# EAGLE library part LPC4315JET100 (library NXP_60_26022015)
32-bit ARM Cortex-M4/M0 MCU; up to 1 MB flash and 136 kB SRAM; Ethernet, two High-speed USB, LCD, EMC The LPC435x/3x/2x/1x are ARM Cortex-M4 based microcontrollers for embedded applications which include an ARM Cortex-M0 coprocessor, up to 1 MB of flash and 136 kB of on-chip SRAM, 16 kB of EEPROM memory, a quad SPI Flash Interface (SPIFI), advanced configurable peripherals such as the State Configurable Timer (SCT) and the Serial General Purpose I/O (SGPIO) interface, two High-speed USB controllers, Ethernet, LCD, an external memory controller, and multiple digital and analog peripherals. The LPC435x/3x/2x/1x operate at CPU frequencies of up to 204 MHz. The ARM Cortex-M4 is a next generation 32-bit core that offers system enhancements such as low power consumption, enhanced debug features, and a high level of support block integration. The ARM Cortex-M4 CPU incorporates a 3-stage pipeline, uses a Harvard architecture with separate local instruction and data buses as well as a third bus for peripherals, and includes an internal prefetch unit that supports speculative branching. The ARM Cortex-M4 supports single-cycle digital signal processing and SIMD instructions. A hardware floating-point unit is integrated in the core. The ARM Cortex-M0 coprocessor is an energy-efficient and easy-to-use 32-bit core which is upward code- and tool-compatible with the Cortex-M4 core. The Cortex-M0 coprocessor, designed as a replacement for existing 8/16-bit microcontrollers, offers up to 204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
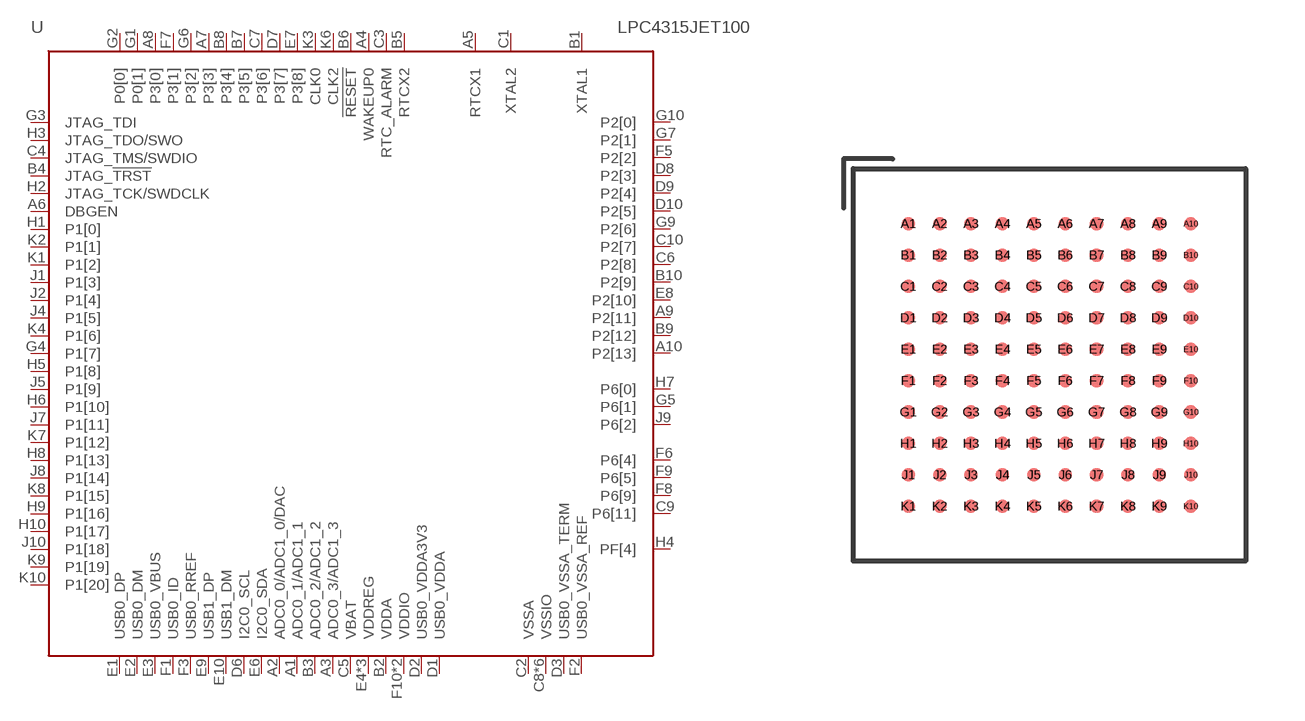
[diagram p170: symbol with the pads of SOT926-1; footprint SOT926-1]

Designator prefix U

## LPC4315JET100  [SOT926-1]
A1  ADC0_1/ADC1_1  in
A2  ADC0_0/ADC1_0/DAC  in
A3  ADC0_3/ADC1_3  in
A4  WAKEUP0  in
A5  RTCX1  in
A6  DBGEN  in
A7  P3[3]
A8  P3[0]
A9  P2[11]
A10  P2[13]
B1  XTAL1  in
B2  VDDA  pwr
B3  ADC0_2/ADC1_2  in
B4  JTAG_!TRST  in
B5  RTCX2  out
B6  !RESET!  in
B7  P3[5]
B8  P3[4]
B9  P2[12]
B10  P2[9]
C1  XTAL2  out
C2  VSSA  pwr
C3  RTC_ALARM  out
C4  JTAG_TMS/SWDIO  in
C5  VBAT  pwr
C6  P2[8]
C7  P3[6]
C8  VSSIO  pwr
C9  P6[11]
C10  P2[7]
D1  USB0_VDDA  pwr
D2  USB0_VDDA3V3  pwr
D3  USB0_VSSA_TERM  pwr
D4  VSSIO  pwr
D5  VSSIO  pwr
D6  I2C0_SCL
D7  P3[7]
D8  P2[3]
D9  P2[4]
D10  P2[5]
E1  USB0_DP
E2  USB0_DM
E3  USB0_VBUS
E4  VDDREG  pwr
E5  VDDREG  pwr
E6  I2C0_SDA
E7  P3[8]
E8  P2[10]
E9  USB1_DP
E10  USB1_DM
F1  USB0_ID  in
F2  USB0_VSSA_REF  pwr
F3  USB0_RREF  pas
F4  VDDREG  pwr
F5  P2[2]
F6  P6[4]
F7  P3[1]
F8  P6[9]
F9  P6[5]
F10  VDDIO  pwr
G1  P0[1]
G2  P0[0]
G3  JTAG_TDI  in
G4  P1[7]
G5  P6[1]
G6  P3[2]
G7  P2[1]
G8  VSSIO  pwr
G9  P2[6]
G10  P2[0]
H1  P1[0]
H2  JTAG_TCK/SWDCLK  in
H3  JTAG_TDO/SWO  out
H4  PF[4]
H5  P1[8]
H6  P1[10]
H7  P6[0]
H8  P1[13]
H9  P1[16]
H10  P1[17]
J1  P1[3]
J2  P1[4]
J3  VSSIO  pwr
J4  P1[5]
J5  P1[9]
J6  VSSIO  pwr
J7  P1[11]
J8  P1[14]
J9  P6[2]
J10  P1[18]
K1  P1[2]
K2  P1[1]
K3  CLK0
K4  P1[6]
K5  VDDIO  pwr
K6  CLK2
K7  P1[12]
K8  P1[15]
K9  P1[19]
K10  P1[20]

## Footprint SOT926-1 (pad centres in mm)
SOT926-1 TFBGA100: plastic thin fine-pitch ball grid array package; 100 balls; body 9 x 9 x 0.7 mm JEDEC: -- IEC: --
smd 0.35 x 0.35: A1 -3.6,3.6; A2 -2.8,3.6; A3 -2,3.6; A4 -1.2,3.6; A5 -0.4,3.6; A6 0.4,3.6; A7 1.2,3.6; A8 2,3.6; A9 2.8,3.6; A10 3.6,3.6; B1 -3.6,2.8; B2 -2.8,2.8; B3 -2,2.8; B4 -1.2,2.8; B5 -0.4,2.8; B6 0.4,2.8; B7 1.2,2.8; B8 2,2.8; B9 2.8,2.8; B10 3.6,2.8; C1 -3.6,2; C2 -2.8,2; C3 -2,2; C4 -1.2,2; C5 -0.4,2; C6 0.4,2; C7 1.2,2; C8 2,2; C9 2.8,2; C10 3.6,2; D1 -3.6,1.2; D2 -2.8,1.2; D3 -2,1.2; D4 -1.2,1.2; D5 -0.4,1.2; D6 0.4,1.2; D7 1.2,1.2; D8 2,1.2; D9 2.8,1.2; D10 3.6,1.2; E1 -3.6,0.4; E2 -2.8,0.4; E3 -2,0.4; E4 -1.2,0.4; E5 -0.4,0.4; E6 0.4,0.4; E7 1.2,0.4; E8 2,0.4; E9 2.8,0.4; E10 3.6,0.4; F1 -3.6,-0.4; F2 -2.8,-0.4; F3 -2,-0.4; F4 -1.2,-0.4; F5 -0.4,-0.4; F6 0.4,-0.4; F7 1.2,-0.4; F8 2,-0.4; F9 2.8,-0.4; F10 3.6,-0.4; G1 -3.6,-1.2; G2 -2.8,-1.2; G3 -2,-1.2; G4 -1.2,-1.2; G5 -0.4,-1.2; G6 0.4,-1.2; G7 1.2,-1.2; G8 2,-1.2; G9 2.8,-1.2; G10 3.6,-1.2; H1 -3.6,-2; H2 -2.8,-2; H3 -2,-2; H4 -1.2,-2; H5 -0.4,-2; H6 0.4,-2; H7 1.2,-2; H8 2,-2; H9 2.8,-2; H10 3.6,-2; J1 -3.6,-2.8; J2 -2.8,-2.8; J3 -2,-2.8; J4 -1.2,-2.8; J5 -0.4,-2.8; J6 0.4,-2.8; J7 1.2,-2.8; J8 2,-2.8; J9 2.8,-2.8; J10 3.6,-2.8; K1 -3.6,-3.6; K2 -2.8,-3.6; K3 -2,-3.6; K4 -1.2,-3.6; K5 -0.4,-3.6; K6 0.4,-3.6; K7 1.2,-3.6; K8 2,-3.6; K9 2.8,-3.6; K10 3.6,-3.6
